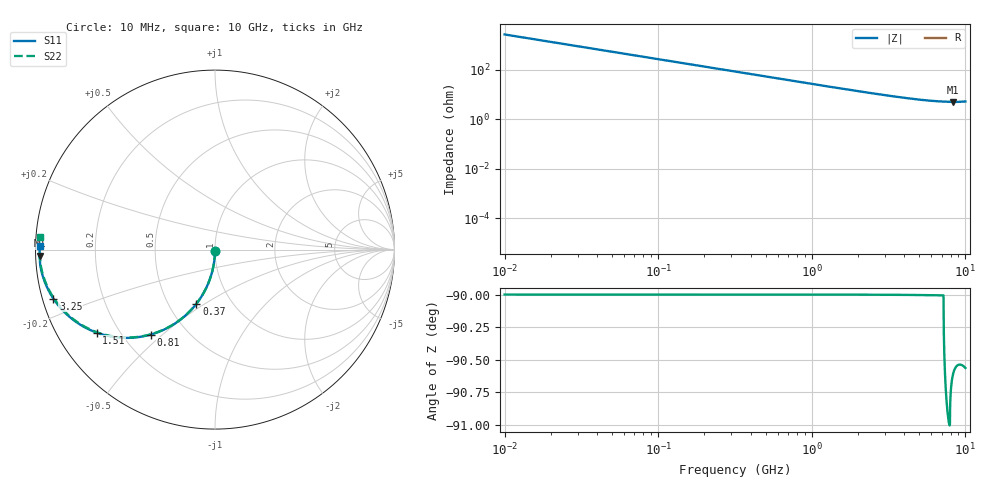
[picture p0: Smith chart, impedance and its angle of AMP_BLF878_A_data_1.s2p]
! Created Tue Mar 09 13:56:48 2010
# ghz S ma R 50
! 2 Port Network Data from SP1.SP block
! freq  magS11  angS11  magS21  angS21  magS12  angS12  magS22  angS22
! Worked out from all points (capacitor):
!   1000 points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, 10 MHz to 10 GHz, reference 50 ohm
!   read as one part in shunt: C = 5.87 pF near 60 MHz
!   lowest |Z| = 5.08 ohm at 8.35 GHz (marker M1)
!   S11 on the Smith chart (normalised r, x): 10 MHz: 1.00, -0.02; 370 MHz: 0.69, -0.46; 810 MHz: 0.31, -0.46; 1.51 GHz: 0.12, -0.31; 3.25 GHz: 0.03, -0.15; 10 GHz: 0.01, +0.01
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0.01  0.00913 -90.5  1 -0.5  1 -0.5  0.00913 -90.5
0.03  0.02738 -91.6  0.9996 -1.6  0.9996 -1.6  0.02738 -91.6
0.08  0.07285 -94.2  0.9973 -4.3  0.9973 -4.3  0.07285 -94.3
0.1  0.09092 -95.3  0.9959 -5.3  0.9959 -5.3  0.09092 -95.3
0.13  0.1179 -96.9  0.993 -6.9  0.993 -6.9  0.1179 -96.9
0.17  0.1534 -99.0  0.9882 -9.0  0.9882 -9.0  0.1534 -99.0
0.23  0.2054 -102.0  0.9787 -12.1  0.9787 -12.1  0.2054 -102.1
0.29  0.2558 -105.1  0.9667 -15.1  0.9667 -15.1  0.2558 -105.1
0.37  0.3198 -109.0  0.9475 -19.0  0.9475 -19.0  0.3198 -109.0
0.56  0.4545 -117.5  0.8907 -27.6  0.8907 -27.6  0.4545 -117.6
0.81  0.593 -127.1  0.8052 -37.1  0.8052 -37.1  0.593 -127.2
1.16  0.7242 -137.4  0.6895 -47.5  0.6895 -47.5  0.7242 -137.6
1.51  0.8056 -145.0  0.5925 -55.1  0.5925 -55.1  0.8056 -145.3
1.68  0.8334 -147.9  0.5527 -58.1  0.5527 -58.1  0.8334 -148.3
2.35  0.9008 -156.3  0.4341 -66.6  0.4341 -66.6  0.9008 -156.8
3.25  0.9411 -163.2  0.338 -73.5  0.338 -73.5  0.9411 -163.9
3.34  0.9436 -163.7  0.331 -74.1  0.331 -74.1  0.9436 -164.4
5.01  0.969 -170.5  0.247 -81.1  0.247 -81.1  0.969 -171.7
6.67  0.9771 -174.8  0.2127 -85.6  0.2127 -85.6  0.9771 -176.4
8.34  0.9774 -178.0  0.2007 -89.7  0.2007 -89.7  0.9775 179.8
8.35  0.9774 -178.0  0.2007 -89.7  0.2007 -89.7  0.9775 179.8
10  0.9755 178.7  0.2104 -93.3  0.2104 -93.3  0.9755 175.9
